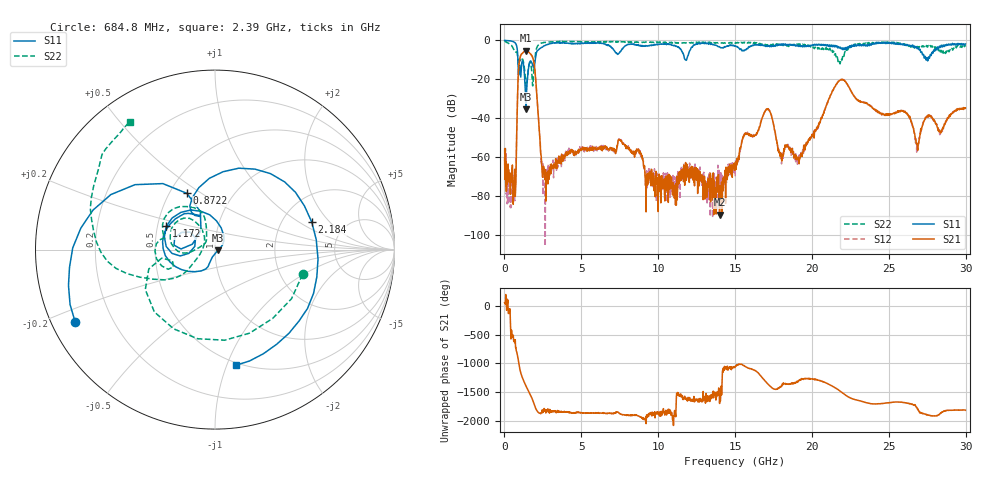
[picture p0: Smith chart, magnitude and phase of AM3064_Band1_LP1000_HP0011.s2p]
# Hz S DB R 50.0
!freq dBS11 angS11 dBS21 angS21 dBS12 angS12 dBS22 angS22
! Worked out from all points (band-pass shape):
!   1600 points, 10 MHz to 29.98 GHz, reference 50 ohm
!   highest |S21| = -5.29 dB at 1.397 GHz (marker M1); lowest = -89.6 dB at 13.99 GHz (marker M2)
!   |S21| within 3 dB of the highest: 1.033 GHz to 1.81 GHz (777.2 MHz wide, 54.7 % of centre)
!   lowest |S11| = -35.4 dB at 1.397 GHz (marker M3), VSWR 1.03, Z = 51.7 - j0.428 ohm
!   |S11| at or under -10 dB: 876.6 MHz to 1.997 GHz (1.12 GHz wide, 78 % of centre); 11.78 GHz to 11.84 GHz (63.31 MHz wide, 0.536 % of centre); 27.50981 GHz to 27.55226 GHz (42.46 MHz wide, 0.154 % of centre)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
!   |S22| runs from -23.6 to -0.3 dB; largest |S21 - S12| = 0.0061
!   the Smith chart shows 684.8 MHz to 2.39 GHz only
!   S11 on the Smith chart (normalised r, x): 684.8 MHz: 0.07, -0.24; 872.2 MHz: 0.61, +0.44; 1.172 GHz: 0.56, +0.16; 2.184 GHz: 2.91, +1.30; 2.39 GHz: 0.48, -1.08
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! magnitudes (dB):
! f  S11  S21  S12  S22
! 10 MHz  0.0  -60.5  -55.5  -0.3
! 309.9 MHz  -0.2  -68.5  -72.6  -1.6
! 684.8 MHz  -1.1  -70.4  -74.5  -5.9
! 872.2 MHz  -9.1  -22.9  -22.9  -10.4
! 1.172 GHz  -10.4  -6.6  -6.5  -9.6
! 1.397 GHz  -35.4  -5.3  -5.3  -22.9
! 1.866 GHz  -13.5  -9.5  -9.4  -21.1
! 2.184 GHz  -5.0  -36.8  -36.8  -2.5
! 2.39 GHz  -3.7  -59.6  -63.5  -1.4
! 2.747 GHz  -2.3  -70.2  -68.7  -0.9
! 5.015 GHz  -1.5  -55.6  -55.6  -0.7
! 7.545 GHz  -5.8  -51.5  -51.4  -0.7
! 10 GHz  -2.0  -88.0  -77.0  -0.9
! 13.99 GHz  -3.3  -89.6  -69.4  -1.2
! 15 GHz  -3.0  -64.6  -69.6  -1.5
! 17.07 GHz  -2.9  -35.6  -35.3  -2.2
! 18 GHz  -2.0  -58.1  -60.0  -2.4
! 19.99 GHz  -2.8  -49.1  -49.2  -3.1
! 21.9 GHz  -4.3  -20.2  -20.0  -9.5
! 25 GHz  -1.1  -38.1  -38.0  -1.1
! 26.85 GHz  -4.2  -53.9  -53.4  -3.1
! 29.98 GHz  -1.8  -34.8  -34.7  -3.2
